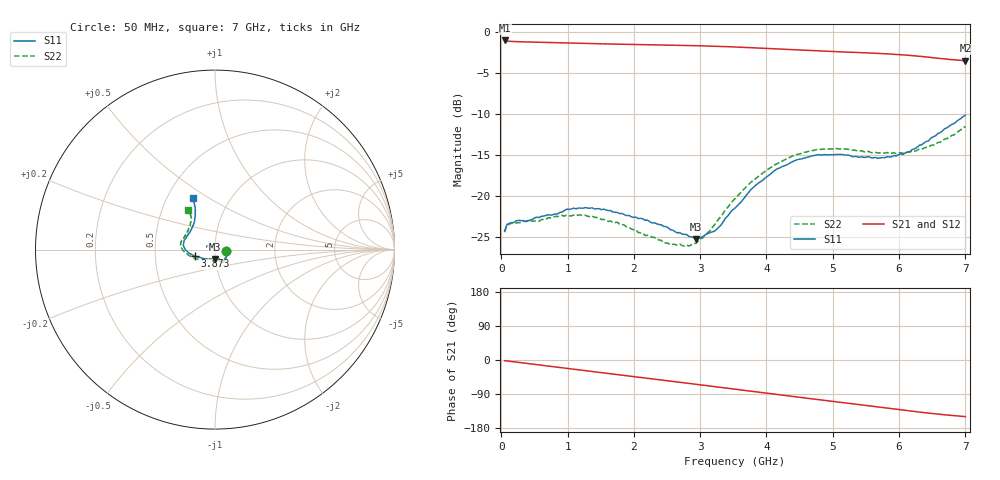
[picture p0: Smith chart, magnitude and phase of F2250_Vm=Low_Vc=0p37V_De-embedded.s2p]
! Integrated Device Technology
! Corporate Headquarters
! 6024 Silver Creek Valley Road
! San Jose, CA 95138  USA
! Phone:  1-408-284-8200
! Toll Free:  1-800-223-1366
! Webpage:  http://www.idt.com/
! Timing and RF Division
! 515 Groton Road, Suite 102
! Westford, MA 01886-6024
! Device:  F2250
! Description: Voltage Variable RF Attenuator
! Frequency:  50.0 -  6000.00 MHz
! Package:  3x3 mm Thin QFN Plastic Package: 16 pin
! Ports:  2 RF, 3 DC
!  Pin  1  = GND
!  Pin  2  = NC
!  Pin  3  = RF1  = Port 1
!  Pin  4  = NC
!  Pin  5  = GND
!  Pin  6  = GND
!  Pin  7  = GND
!  Pin  8  = GND
!  Pin  9  = NC
!  Pin 10  = RF2  = Port 2
!  Pin 11  = NC
!  Pin 12  = GND
!  Pin 13  = GND
!  Pin 14  = VCNTRL
!  Pin 15  = VDD
!  Pin 16  = VMODE
! Vcntrl:  0.370 Volts
! Vmode:  +0.000 Volts
! Vdd:  +3.30  Volts
! Current:  1.121 mA
! Data:  The device was measured on a the F2250 evaluation board which has
!  individual transmission lines to the RF pins.  Data was collected
!  using a calibrated network analyzer.  The evaluation board was
!  de-embedded using a TRL calibration technique.
!  The reference plane is the edge of the package pin.
! Misc:  SN 10
!  Action Tracker AT0258
! Date Measured:  2014-11-26
! Date:  2015-10-15  MJV
! Note:
!  Integrated Device Technology supplies this data as a sample of measured
!  data at the package pin for this product.  Your particular data for this
!  product may vary.
!  Data was taken at 25 degrees C.
!  Integrated Device Technology reserves the right to change this data at anytime.
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# GHz S dB R 50
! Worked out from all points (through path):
!   201 points, 50 MHz to 7 GHz, reference 50 ohm
!   highest |S21| = -0.98 dB at 50 MHz (marker M1); lowest = -3.5 dB at 7 GHz (marker M2)
!   group delay of S21, straight-line fit = 60 ps
!   lowest |S11| = -25.3 dB at 2.934 GHz (marker M3), VSWR 1.12, Z = 49.9 - j5.45 ohm
!   |S11| at or under -10 dB: start of sweep to end of sweep
!   |S22| runs from -26.2 to -11.5 dB; largest |S21 - S12| = 0.00034
!   S11 on the Smith chart (normalised r, x): 50 MHz: 1.13, -0.02; 3.873 GHz: 0.79, -0.06; 7 GHz: 0.67, +0.42
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0.05  -24.33 -8.9  -0.98 -1.8  -0.98 -1.8  -24.46 -9.5
0.08475  -23.52 -8.9  -1.05 -2.5  -1.05 -2.5  -23.61 -8.8
0.15425  -23.29 -11.1  -1.10 -4.0  -1.09 -4.0  -23.37 -10.6
0.57125  -22.67 -28.4  -1.20 -13.1  -1.20 -13.1  -23.11 -29.5
0.884  -22.04 -43.6  -1.26 -20.0  -1.26 -19.9  -22.42 -45.5
1.2315  -21.53 -53.6  -1.34 -27.4  -1.34 -27.4  -22.44 -58.3
1.75275  -22.05 -60.3  -1.43 -38.4  -1.43 -38.4  -23.24 -65.9
2.37825  -23.52 -61.4  -1.52 -51.8  -1.52 -51.8  -25.42 -68.9
2.552  -24.16 -65.3  -1.55 -55.6  -1.55 -55.6  -26.03 -74.6
2.83  -24.98 -79.5  -1.60 -61.7  -1.60 -61.7  -26.16 -92.9
2.93425  -25.28 -88.0  -1.62 -64.0  -1.62 -64.0  -25.84 -101.3
3.21225  -24.36 -117.0  -1.68 -70.2  -1.68 -70.2  -23.57 -126.4
3.525  -21.52 -144.5  -1.78 -77.1  -1.78 -77.1  -20.36 -145.3
3.8725  -18.47 -161.7  -1.91 -84.8  -1.91 -84.8  -17.66 -160.7
4.1505  -16.75 -171.7  -2.02 -90.9  -2.02 -90.9  -16.10 -170.7
4.4285  -15.70 -179.4  -2.13 -96.9  -2.13 -96.9  -15.02 -177.9
4.7065  -15.10 173.8  -2.23 -102.9  -2.23 -102.9  -14.46 176.0
5.15825  -14.96 163.0  -2.39 -112.6  -2.39 -112.6  -14.22 166.8
5.85325  -15.26 139.7  -2.64 -127.6  -2.64 -127.6  -14.82 151.6
6.166  -14.58 128.6  -2.81 -134.4  -2.81 -134.4  -14.65 142.7
6.444  -13.26 120.1  -3.02 -140.2  -3.02 -140.2  -14.05 133.3
7  -10.14 113.6  -3.46 -149.4  -3.46 -149.5  -11.52 123.8
